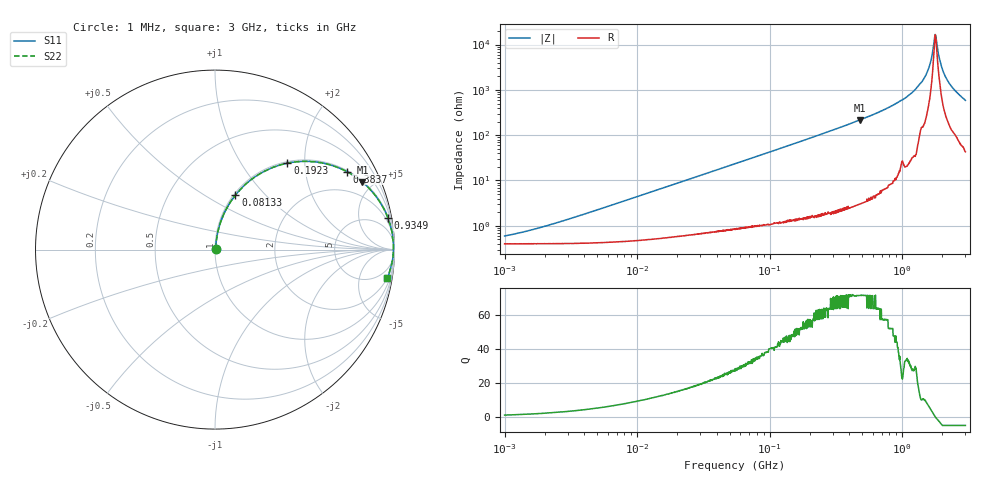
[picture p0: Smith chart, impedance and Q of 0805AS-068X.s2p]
!s-Parameter Generated by FASTRON Sdn. Bhd.
!FASTRON P/N : 0805AS-068X
!Keysight Technologies: E4991B_MY54100416_A.01.15
!Date: Mon Jun 15 12:51:27 2026
!Version  :Rev01  Mon Jun 15 12:51:27 2026
!Data & Calibration Information:
!Freq  S11  S21  S12  S22
!PortZ  Port1:50+j0  Port2:50+j0
!When reading reference impedance value at option line is always used.
! Remarks : This data is being provided solely for informational purposes.
# Hz S dB R 50
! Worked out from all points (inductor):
!   1601 points, 1 MHz to 3 GHz, reference 50 ohm
!   read as one part in series: L = 70.5 nH near 2.748 MHz
!   highest Q = 71.6 at 480.5 MHz (marker M1), where L = 71.8 nH
!   self-resonance near 1.774 GHz
!   S11 on the Smith chart (normalised r, x): 1 MHz: 1.01, +0.01; 81.33 MHz: 1.02, +0.69; 192.3 MHz: 1.03, +1.64; 383.7 MHz: 1.04, +3.37; 934.9 MHz: 1, +11; 3 GHz: 2, -12
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1000000  -44.50 47.6  -0.03 -0.3  -0.03 -0.3  -44.50 47.6
3804036  -35.30 75.3  -0.04 -1.0  -0.04 -1.0  -35.30 75.3
1.447069e7  -24.00 81.7  -0.06 -3.6  -0.06 -3.6  -24.00 81.7
5.504702e7  -12.90 74.8  -0.30 -13.1  -0.30 -13.1  -12.90 74.8
8.132864e7  -9.78 69.4  -0.57 -18.9  -0.57 -18.9  -9.78 69.4
1.923242e8  -4.04 50.0  -2.31 -38.9  -2.31 -38.9  -4.04 50.0
2.083556e8  -3.63 47.8  -2.61 -41.2  -2.61 -41.2  -3.63 47.8
3.836505e8  -1.36 30.5  -5.90 -58.7  -5.90 -58.7  -1.36 30.5
4.805402e8  -0.89 24.6  -7.60 -64.6  -7.60 -64.6  -0.89 24.6
7.925923e8  -0.29 13.6  -12.60 -75.3  -12.60 -75.3  -0.29 13.6
9.349007e8  -0.19 10.5  -14.80 -78.0  -14.80 -78.0  -0.19 10.5
1.206698e9  -0.09 6.2  -19.30 -81.7  -19.30 -81.7  -0.09 6.2
1.45942e9  -0.06 3.2  -25.00 -81.2  -25.00 -81.2  -0.06 3.2
1.596974e9  -0.05 1.8  -30.10 -78.6  -30.10 -78.6  -0.05 1.8
1.653904e9  -0.05 1.2  -33.30 -74.8  -33.30 -74.8  -0.05 1.2
1.730092e9  -0.05 0.5  -40.10 -55.1  -40.10 -55.1  -0.05 0.5
1.782824e9  -0.05 -0.0  -44.30 3.8  -44.30 3.8  -0.05 -0.0
1.827992e9  -0.06 -0.4  -40.20 47.7  -40.20 47.7  -0.06 -0.4
1.970482e9  -0.06 -1.6  -30.80 75.3  -30.80 75.3  -0.06 -1.6
2.145442e9  -0.08 -3.1  -25.30 79.0  -25.30 79.0  -0.08 -3.1
2.455801e9  -0.13 -5.5  -20.40 78.4  -20.40 78.4  -0.13 -5.5
3e9  -0.23 -9.5  -15.60 76.3  -15.60 76.3  -0.23 -9.5
